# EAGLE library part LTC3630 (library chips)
65 V 500 mA Step Down converter
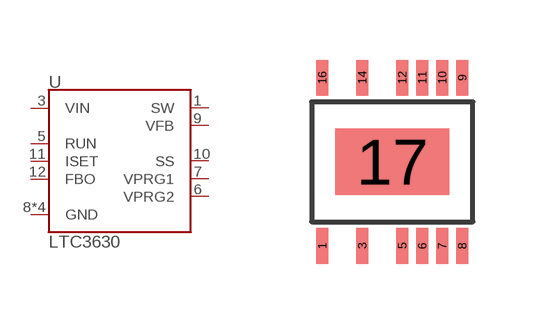
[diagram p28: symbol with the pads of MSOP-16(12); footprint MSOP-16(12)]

Designator prefix U

## LTC3630 (DIGIKEY: LTC3630EMSE#PBF-ND)  [MSOP-16(12)]
1  SW
3  VIN
5  RUN
6  VPRG2
7  VPRG1
8  GND
9  VFB
10  SS
11  ISET
12  FBO
14  GND
16  GND
17  GND

## Footprint MSOP-16(12) (pad centres in mm)
smd 0.305 x 0.889: 1 -1.75,-2.106; 3 -0.75,-2.106; 5 0.25,-2.106; 6 0.75,-2.106; 7 1.25,-2.106; 8 1.75,-2.106; 9 1.75,2.106; 10 1.25,2.106; 11 0.75,2.106; 12 0.25,2.106; 14 -0.75,2.106; 16 -1.75,2.106
smd 2.845 x 1.651: 17 0,0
